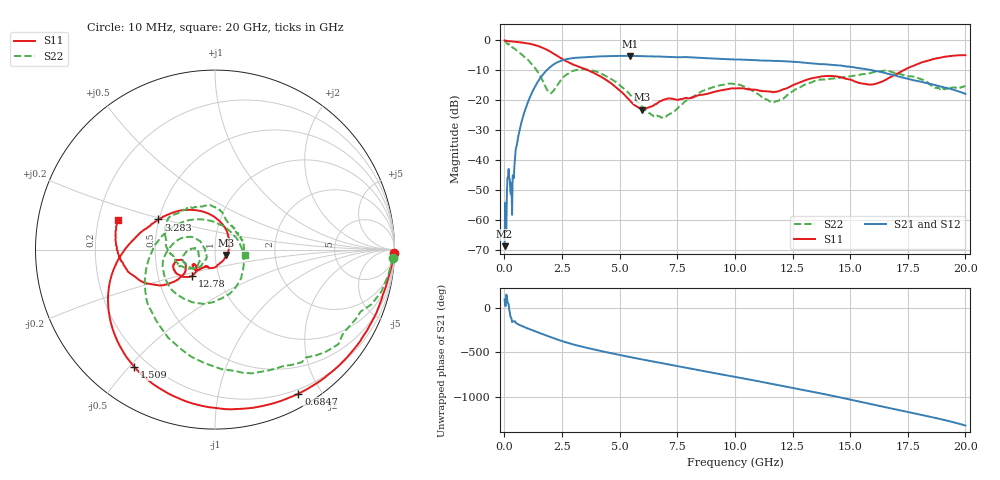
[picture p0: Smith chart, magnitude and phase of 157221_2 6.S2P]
!  2-Port S-parameters saved by WinCal
! VAR MeasName=S-Parameters (CALIBRATED_DATA) read from VNA (N5242A)
! VAR MeasDate=2015-5-26 16:47:37
! VAR NAME=157221_2 6
! VAR FILENAME=157221_2 6.S2P
! VAR DATE=2015-5-26 16:47:37
! VAR PHYS_PORTS=1,2
# Hz S DB R 50
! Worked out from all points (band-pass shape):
!   801 points, 10 MHz to 20 GHz, reference 50 ohm
!   highest |S21| = -5.18 dB at 5.457 GHz (marker M1); lowest = -68.7 dB at 10 MHz (marker M2)
!   |S21| within 3 dB of the highest: 2.111 GHz to 14.18 GHz (12.07 GHz wide, 148 % of centre); 14.17933 GHz to 14.21687 GHz (37.53 MHz wide, 0.264 % of centre)
!   lowest |S11| = -23.2 dB at 5.982 GHz (marker M3), VSWR 1.15, Z = 56.6 - j3.35 ohm
!   |S11| at or under -10 dB: 3.627 GHz to 17.31 GHz (13.68 GHz wide, 131 % of centre)
!   |S22| runs from -25.9 to -0.1 dB; largest |S21 - S12| = 0.0078
!   S11 on the Smith chart (normalised r, x): 10 MHz: open; 684.7 MHz: 0.15, -1.72; 1.509 GHz: 0.15, -0.52; 3.283 GHz: 0.50, +0.19; 12.78 GHz: 0.74, -0.23; 20 GHz: 0.28, +0.14
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1e7  -0.04 -1.1  -68.65 98.4  -70.40 27.4  -0.06 -2.6
1.349375e8  -0.24 -12.9  -45.80 72.1  -46.08 70.1  -1.16 -26.1
3.59825e8  -0.39 -32.4  -45.08 -147.3  -44.97 -147.3  -2.49 -60.2
6.846625e8  -0.65 -60.0  -29.22 166.0  -29.21 166.0  -4.27 -102.4
1.084462e9  -1.13 -92.4  -19.39 122.3  -19.37 122.2  -7.03 -151.0
1.50925e9  -2.01 -124.5  -13.09 80.0  -13.07 79.8  -11.33 154.1
2.258875e9  -5.03 -171.2  -7.47 7.9  -7.46 7.6  -15.37 -19.5
3.283362e9  -8.92 152.0  -5.74 -71.3  -5.75 -71.6  -9.76 -125.9
3.358325e9  -9.18 149.4  -5.68 -76.2  -5.70 -76.4  -9.69 -130.9
4.50775e9  -13.67 101.5  -5.28 -143.5  -5.28 -143.6  -12.37 173.8
5.457275e9  -20.20 37.5  -5.18 165.6  -5.17 165.4  -18.16 150.2
5.982012e9  -23.16 -25.1  -5.26 138.4  -5.26 138.3  -22.14 157.1
6.681662e9  -20.69 -83.6  -5.38 103.3  -5.36 103.3  -25.39 -167.4
8.430788e9  -18.30 -123.6  -5.80 17.7  -5.80 17.4  -17.65 -130.9
1.0005e10  -15.97 -136.6  -6.38 -57.8  -6.38 -58.3  -14.57 -164.2
1.162919e10  -17.17 -139.9  -6.83 -137.3  -6.79 -137.9  -20.53 -170.9
1.277861e10  -14.14 -131.2  -7.28 163.4  -7.29 163.1  -15.77 -139.3
1.335332e10  -12.63 -139.6  -7.69 133.8  -7.65 133.6  -13.91 -151.5
1.525238e10  -13.89 -163.6  -9.12 31.0  -9.01 30.7  -11.74 -178.7
1.667666e10  -12.59 -141.6  -11.21 -49.6  -11.16 -49.8  -10.24 143.1
1.842579e10  -6.68 -159.9  -14.45 -146.4  -14.38 -147.7  -14.47 73.4
2e10  -4.96 162.9  -17.87 112.6  -17.96 110.8  -15.30 -9.2
